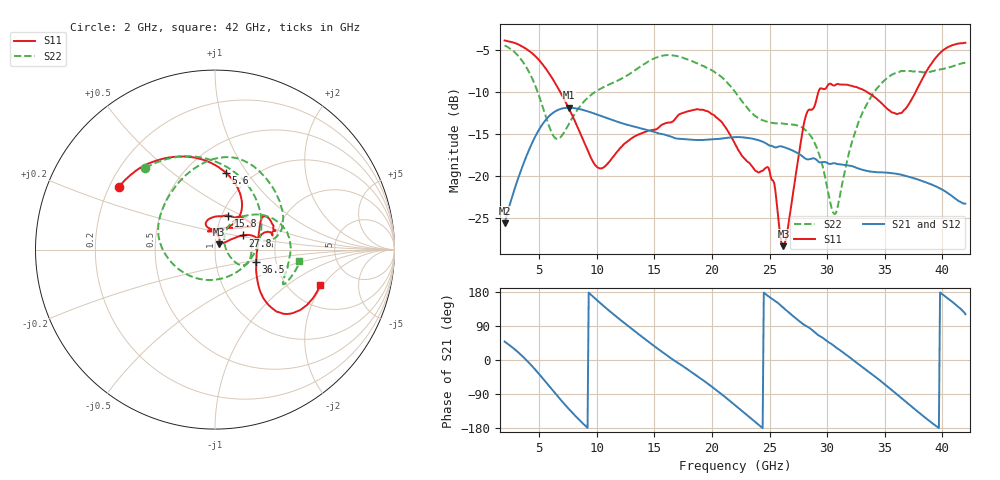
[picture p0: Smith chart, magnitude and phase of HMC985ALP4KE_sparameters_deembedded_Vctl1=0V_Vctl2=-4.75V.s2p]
!s2p File: Measurements: S11, S21, S12, S22
# GHz S dB R 50.0
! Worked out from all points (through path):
!   401 points, 2 GHz to 42 GHz, reference 50 ohm
!   highest |S21| = -11.90 dB at 7.6 GHz (marker M1); lowest = -25.7 dB at 2 GHz (marker M2)
!   lowest |S11| = -28.4 dB at 26.2 GHz (marker M3), VSWR 1.08, Z = 52.3 + j3.17 ohm
!   |S11| at or under -10 dB: 6.82 GHz to 29.25 GHz (22.43 GHz wide, 124 % of centre); 33.42 GHz to 37.69 GHz (4.268 GHz wide, 12 % of centre)
!   |S22| runs from -24.6 to -4.5 dB; largest |S21 - S12| = 0.00021
!   S11 on the Smith chart (normalised r, x): 2 GHz: 0.24, +0.28; 5.6 GHz: 0.76, +0.80; 15.8 GHz: 1.07, +0.42; 27.8 GHz: 1.34, +0.22; 36.5 GHz: 1.57, -0.23; 42 GHz: 2.94, -1.89
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2  -3.88 147.0  -25.67 48.6  -25.67 48.6  -4.47 130.5
3.6  -4.66 120.3  -18.70 8.4  -18.70 8.4  -6.47 84.9
4.7  -5.80 99.5  -15.22 -26.8  -15.22 -26.8  -9.41 43.4
5.6  -7.29 81.9  -13.30 -59.0  -13.30 -59.0  -13.04 -3.7
6.5  -9.22 66.5  -12.25 -91.9  -12.25 -91.9  -15.60 -68.8
7.6  -12.04 54.8  -11.90 -130.0  -11.90 -130.1  -13.77 -135.6
8.7  -15.38 55.1  -12.12 -164.6  -12.12 -164.7  -11.46 -170.1
10.4  -19.13 89.6  -12.90 147.6  -12.90 147.6  -9.58 162.5
15.4  -14.23 75.7  -14.97 27.6  -14.97 27.6  -5.81 87.3
15.8  -13.84 68.7  -15.07 18.7  -15.07 18.7  -5.67 82.2
19.4  -12.23 33.3  -15.73 -57.1  -15.73 -57.1  -7.03 35.2
22  -16.18 51.1  -15.40 -119.2  -15.41 -119.2  -10.00 9.8
24.9  -19.04 104.8  -16.33 168.1  -16.33 168.1  -13.60 13.2
26.2  -28.39 52.8  -16.57 137.7  -16.57 137.7  -13.79 -2.3
27.8  -15.23 27.2  -17.63 97.2  -17.64 97.2  -14.22 -24.1
28.7  -12.11 12.6  -17.92 79.1  -17.93 79.1  -15.51 -31.2
30.7  -9.21 20.7  -18.53 34.8  -18.53 34.8  -24.56 21.1
32.8  -9.59 33.9  -19.17 -12.8  -19.18 -12.8  -13.33 53.6
35.4  -12.21 11.8  -19.66 -74.0  -19.66 -74.0  -8.18 21.7
36.5  -12.48 -16.7  -19.90 -101.8  -19.91 -101.9  -7.53 7.6
39.5  -5.85 -43.8  -21.31 -175.2  -21.31 -175.2  -7.43 -26.4
42  -4.15 -18.6  -23.33 120.8  -23.33 120.8  -6.49 -7.4
